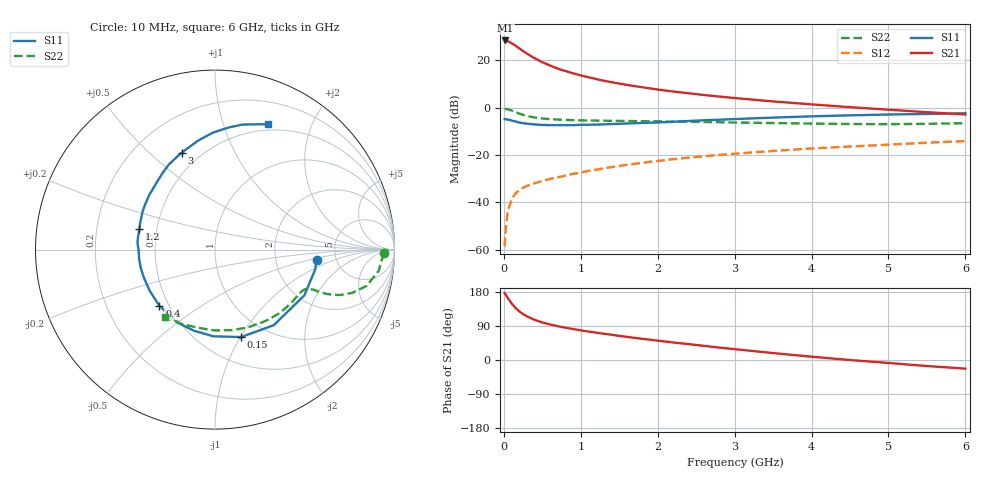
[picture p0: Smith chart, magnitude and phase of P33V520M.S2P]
! SIEMENS Small Signal Semiconductors
! BFP181
! Si NPN RF Bipolar Junction Transistor in SOT143
! VCE = 3.5 V  IC = 20 mA
! Common Emitter S-Parameters:  March  1996
# GHz  S  MA  R  50
!  f  S11  S21  S12  S22
! GHz  MAG  ANG  MAG  ANG  MAG  ANG  MAG  ANG
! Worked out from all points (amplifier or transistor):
!   36 points, 10 MHz to 6 GHz, reference 50 ohm
!   highest |S21| = 28.3 dB at 20 MHz (marker M1)
!   |S21| within 3 dB of that: start of sweep to 186.7 MHz
!   unconditionally stable (mu >= 1): start of sweep to 14.8 MHz; 531.5 MHz to end of sweep
!   at 250 MHz: K = 0.62, MSG = 28.8 dB, |S12| = -33.8 dB
!   at 1.4 GHz: K = 1.38, MAG = 14.2 dB, |S12| = -25.1 dB
!   at 6 GHz: K = 1.08, MAG = 3.9 dB, |S12| = -14.1 dB
!   S11 on the Smith chart (normalised r, x): 10 MHz: 3.53, -0.58; 150 MHz: 0.77, -1.01; 400 MHz: 0.44, -0.35; 1.2 GHz: 0.40, +0.12; 3 GHz: 0.40, +0.64; 6 GHz: 0.43, +1.42
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0.01  0.5687 -5.6  25.86 176.4  0.0012 81.0  0.9391 -1.1
0.02  0.5691 -11.2  25.91 173.6  0.0023 78.3  0.9336 -2.8
0.05  0.5594 -27.1  25.15 164.0  0.0065 82.3  0.9193 -7.4
0.1  0.5334 -52.1  22.74 149.8  0.0115 68.7  0.868 -13.5
0.15  0.5085 -73.4  20.16 137.7  0.0154 60.5  0.8013 -17.5
0.2  0.4831 -91.0  17.72 128.5  0.0182 57.6  0.7459 -19.8
0.25  0.4669 -104.7  15.44 121.0  0.0205 54.7  0.7002 -21.1
0.3  0.4572 -116.7  13.66 115.4  0.0223 53.4  0.6644 -21.7
0.4  0.4408 -134.7  10.95 106.0  0.0254 52.5  0.6166 -22.1
0.5  0.43 -147.9  9.015 99.2  0.0284 51.9  0.588 -22.2
0.6  0.4259 -157.9  7.69 93.8  0.0314 53.0  0.5697 -22.6
0.7  0.4261 -166.0  6.614 89.2  0.0339 54.4  0.5575 -23.1
0.9  0.4257 -179.5  5.268 81.8  0.0401 55.7  0.5426 -24.4
1.1  0.4349 169.5  4.348 74.9  0.0463 56.2  0.533 -26.5
1.2  0.4368 164.4  3.987 72.2  0.049 56.4  0.531 -27.7
1.7  0.4672 144.6  2.823 58.4  0.0653 56.1  0.5185 -34.5
2.2  0.5011 129.1  2.177 46.3  0.0815 53.8  0.5066 -42.4
3  0.5714 108.9  1.587 28.6  0.1064 48.4  0.4832 -56.8
3.5  0.6141 98.9  1.345 18.3  0.1217 44.8  0.4711 -67.0
4.5  0.6849 83.5  1.018 -0.1  0.1507 36.8  0.45 -90.3
5.5  0.7327 72.3  0.798 -15.9  0.1817 29.0  0.454 -114.5
6  0.7579 67.1  0.716 -22.8  0.1965 24.6  0.4678 -126.5
